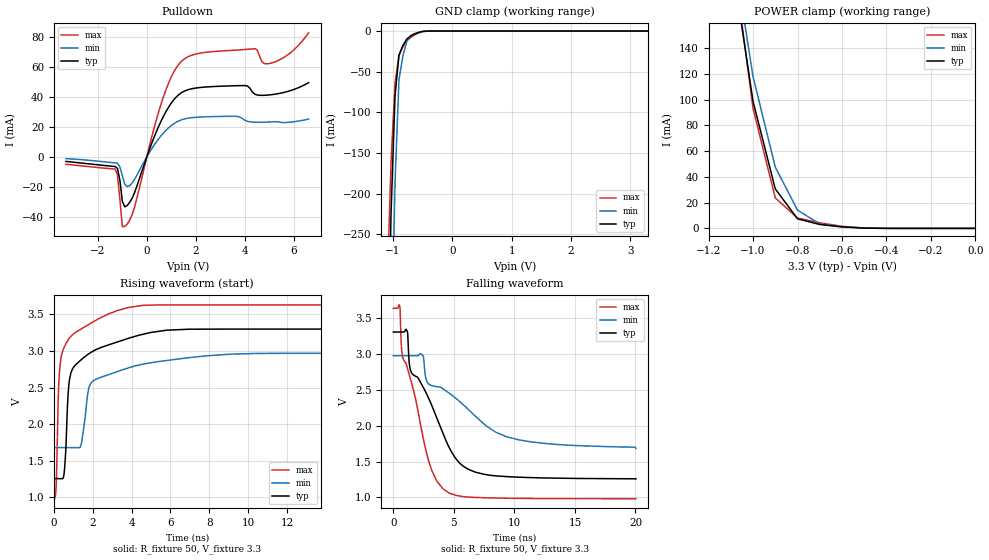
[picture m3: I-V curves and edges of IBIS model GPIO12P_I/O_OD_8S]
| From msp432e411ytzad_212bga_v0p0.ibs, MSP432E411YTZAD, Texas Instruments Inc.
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|   Model Cell GPIO12P_I/O_OD_8S
[Model]   GPIO12P_I/O_OD_8S
Model_type   I/O_open_drain
Polarity   Inverting
Enable   Active-Low
Vinl =  0.8
Vinh =  2
Cref =  15.0000pF
Rref =  100.0000M
Vref =  0V
Vmeas =  1.65
C_comp   6.029616p   5.226915p   6.778838p
[Model Spec]
Vinl   0.8   0.8   0.8
Vinh   2   2   2
[Temperature Range]   25   125   -40
[Voltage Range]   3.3   2.97   3.63
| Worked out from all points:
|   slope of the pulldown table from 0 to 0.495 V, typ, clamps not added: 23.8 ohm
|   GND clamp passes 1 mA (typ) near -0.53 V on its own axis
|   POWER clamp passes 1 mA (typ) near -0.58 V on its own axis
|   rising waveform, R_fixture 50, V_fixture 3.3: 20-80 % time 834ps typ, 1.66ns min, 464ps max; typ from 1.26 V to 3.3 V
|   falling waveform, R_fixture 50, V_fixture 3.3: 20-80 % time 3.4ns typ, 5.55ns min, 2.25ns max; typ from 3.3 V to 1.26 V
| Nom Voltages:
|   IBIASFET=3.3, VDDC=1.2, VDD=3.3, GND=0
| Min Voltages:
|   IBIASFET=2.97, VDDC=1.08, VDD=2.97, GND=0
| Max Voltages:
|   IBIASFET=3.63, VDDC=1.32, VDD=3.63, GND=0
[POWER_clamp]
|   voltage   I(typ)   I(min)   I(max)
-3.3V     3.668A     4.187A     4.057A
-1.067V   175.6mA    191.7mA    181.3mA
-1.033V   137.2mA    154.7mA    137.2mA
-1V       98.66mA    117.8mA    93.17mA
-900mV    30.66mA    47.6mA     23.68mA
-800mV    7.454mA    14.17mA    8.045mA
-700mV    3.021mA    3.466mA    4.326mA
-600mV    1.166mA    1.15mA     1.613mA
-500mV    219.7uA    295.1uA    245.5uA
0V        69.04pA    1.982nA    9.028pA
[Pulldown]
|   voltage   I(typ)   I(min)   I(max)
-3.3V     -3.019mA   -1.206mA   -4.938mA
-1.3V     -6.416mA   -4.007mA   -8.087mA
-1.2V     -7.65mA    -4.163mA   -11.69mA
-1V       -29.59mA   -12.56mA   -46.46mA
-900mV    -33.29mA   -18.21mA   -46.32mA
-500mV    -23.81mA   -14.98mA   -33.54mA
700mV     27.72mA    16.29mA    41.06mA
1.4V      42.61mA    24.62mA    63.44mA
4V        47.51mA    24.37mA    71.53mA
4.4V      41.79mA    23.1mA     72.14mA
5V        41.27mA    23.24mA    62.2mA
6.6V      49.45mA    25.19mA    82.65mA
[GND_clamp]
|   voltage   I(typ)   I(min)   I(max)
-3.3V     -18.01A    -17.27A    -18.6A
-1.1V     -459.9mA   -734.3mA   -318.7mA
-1.033V   -223.6mA   -411.6mA   -160.4mA
-966.7mV  -80.12mA   -186.8mA   -64.21mA
-900mV    -29.51mA   -59.8mA    -30.11mA
-833.3mV  -17.66mA   -30.4mA    -19.41mA
-766.7mV  -9.785mA   -12.28mA   -11.96mA
-700mV    -5.884mA   -5.445mA   -7.749mA
-500mV    -484.3uA   -573uA     -552.3uA
-366.7mV  -23.48uA   -48.41uA   -21.82uA
3.3V      69.03pA    6.412uA    7.794pA
[Ramp]
| variable   typ   min   max
dV/dt_f  1.2484834/3.3898513n 0.79075867/5.5201485n  1.6167624/2.2426289n
dV/dt_r  1.2448904/3.2567253n 0.88403346/5.4513958n  1.5995284/2.1976543n
R_load = 50
[Rising Waveform]
R_fixture = 50
V_fixture = 3.3
V_fixture_min = 2.97
V_fixture_max = 3.63
|   time   V(typ)   V(min)   V(max)
0s        1.258V     1.681V     982.5mV
112.1ps   1.258V     1.681V     1.123V
249ps     1.258V     1.681V     2.527V
410.6ps   1.256V     1.681V     2.957V
550.4ps   1.382V     1.681V     3.061V
880.4ps   2.702V     1.681V     3.202V
1.389ns   2.877V     1.707V     3.299V
1.811ns   2.965V     2.5V       3.366V
2.361ns   3.041V     2.635V     3.449V
20.04ns   3.3V       2.97V      3.63V
[Falling Waveform]
R_fixture = 50
V_fixture = 3.3
V_fixture_min = 2.97
V_fixture_max = 3.63
|   time   V(typ)   V(min)   V(max)
0s        3.3V       2.97V      3.63V
536.6ps   3.3V       2.97V      3.649V
710.7ps   3.3V       2.97V      3.017V
1.152ns   3.31V      2.97V      2.806V
1.45ns    2.753V     2.97V      2.631V
2.471ns   2.533V     2.968V     1.821V
2.918ns   2.381V     2.578V     1.508V
4.094ns   1.897V     2.512V     1.121V
7.391ns   1.325V     2.037V     996.4mV
20.04ns   1.258V     1.681V     982.8mV
